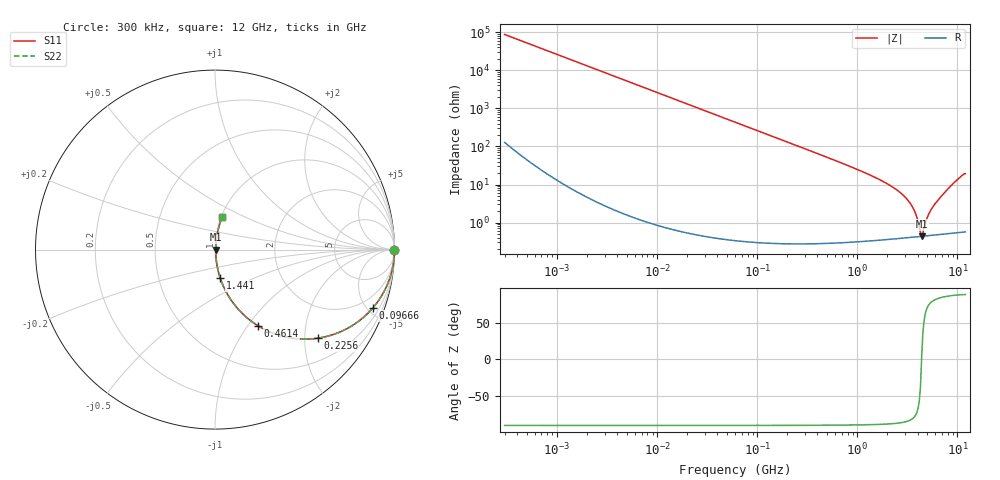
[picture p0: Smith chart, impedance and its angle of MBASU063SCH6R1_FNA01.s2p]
! MBASU063SCH6R1_FNA01  S-PARAMETER MODEL  ( General Type )
! Model Generated by TAIYO YUDEN Corporation (http://www.ty-top.com)
! Version 1.0
! TAIYO YUDEN Control No. 130801
! Copyright(c) 2013 TAIYO YUDEN CO.,LTD. All Rights Reserved.
! Product Description (link to TY-COMPAS)
! https://ds.yuden.co.jp/TYCOMPAS/or/detail?pn=MBASU063SCH6R1DFNA01&u=M
! Products Name : Multilayer Ceramic Capacitors
! Characteristics :
!  Capacitance : 6.1 pF , Rated Voltage : 50V , TCC : CH / C0H
!  Case Size : 0.6 x 0.3 / 0.024 x 0.012 [mm/inch] , Thickness : 0.3 / 0.012 [mm/inch]
!  (Conditions: Temperature = 25 degC , DC Bias Current/Voltage = 0A / 0V)
! External Node Assignments :
!  1  o---| |---o  2
! GND o---------o GND
! Frequency Range : 0.3MHz  -  12000MHz  [ 401 STEP ]
# MHz S RI R 50
! Freq[MHz].  S11 Real  S11 Imag  S21 Real  S21 Imag  S12 Real  S12 Imag  S22 Real  S22 Imag
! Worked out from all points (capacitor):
!   401 points, 300 kHz to 12 GHz, reference 50 ohm
!   read as one part in series: C = 6.07 pF near 316.3 kHz
!   lowest |Z| = 436 mohm at 4.385 GHz (marker M1)
!   series resonance near 4.383 GHz, so ESL is about 220 pH
!   S11 on the Smith chart (normalised r, x): 300 kHz: open; 96.66 MHz: 1.01, -5.42; 225.6 MHz: 1.01, -2.32; 461.4 MHz: 1.01, -1.12; 1.441 GHz: 1.01, -0.32; 12 GHz: 1.01, +0.39
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0.3  1 -0.00114  2.98e-06 0.00114  2.98e-06 0.00114  1 -0.00114
1.769972  1 -0.00675  4.81e-05 0.00675  4.81e-05 0.00675  1 -0.00675
10.44266  0.9984 -0.0398  0.0016 0.0398  0.0016 0.0398  0.9984 -0.0398
27.82928  0.9888 -0.105  0.0112 0.105  0.0112 0.105  0.9888 -0.105
60  0.9501 -0.2174  0.0499 0.2174  0.0499 0.2174  0.9501 -0.2174
96.65937  0.8799 -0.3245  0.1201 0.3245  0.1201 0.3245  0.8799 -0.3245
225.6362  0.573 -0.4935  0.427 0.4935  0.427 0.4935  0.573 -0.4935
353.9943  0.3517 -0.4756  0.6483 0.4756  0.6483 0.4756  0.3517 -0.4756
461.3684  0.2411 -0.4252  0.7589 0.4252  0.7589 0.4252  0.2411 -0.4252
763.2128  0.102 -0.2982  0.898 0.2982  0.898 0.2982  0.102 -0.2982
1441.349  0.0287 -0.1571  0.9713 0.1571  0.9713 0.1571  0.0287 -0.1571
2088.533  0.0129 -0.0955  0.9871 0.0955  0.9871 0.0955  0.0129 -0.0955
2795.104  0.00694 -0.0552  0.9931 0.0552  0.9931 0.0552  0.00694 -0.0552
3364.605  0.00507 -0.0319  0.9949 0.0319  0.9949 0.0319  0.00507 -0.0319
3740.715  0.00453 -0.019  0.9955 0.019  0.9955 0.019  0.00453 -0.019
4158.869  0.00432 -0.00642  0.9957 0.00642  0.9957 0.00642  0.00432 -0.00642
4385.161  0.00434 7.48e-05  0.9957 -7.48e-05  0.9957 -7.48e-05  0.00434 7.48e-05
4623.766  0.00443 0.0053  0.9956 -0.0053  0.9956 -0.0053  0.00443 0.0053
5278.635  0.00488 0.0179  0.9951 -0.0179  0.9951 -0.0179  0.00488 0.0179
6026.253  0.00571 0.0314  0.9943 -0.0314  0.9943 -0.0314  0.00571 0.0314
9207.246  0.0172 0.1081  0.9828 -0.1081  0.9828 -0.1081  0.0172 0.1081
12000  0.0408 0.1836  0.9592 -0.1836  0.9592 -0.1836  0.0408 0.1836
